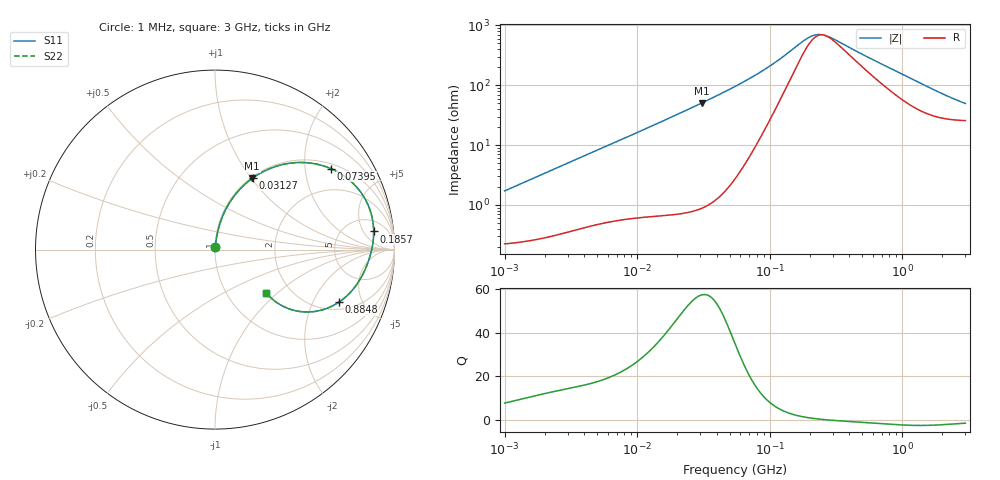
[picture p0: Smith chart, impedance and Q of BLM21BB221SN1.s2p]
! BLM21BB221SN1
# Hz S RI R 50
!Freq.(Hz) S11(Real) S11(Imag) S21(Real) S21(Imag) S12(Real) S12(Imag) S22(Real) S22(Imag)
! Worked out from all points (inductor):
!   401 points, 1 MHz to 3 GHz, reference 50 ohm
!   read as one part in series: L = 270 nH near 1.041 MHz
!   highest Q = 57.5 at 30.65 MHz (marker M1), where L = 262 nH
!   self-resonance near 257.1 MHz
!   S11 on the Smith chart (normalised r, x): 1 MHz: 1.00, +0.03; 31.27 MHz: 1.02, +1.03; 73.95 MHz: 1.15, +2.75; 185.7 MHz: 9, +9; 884.8 MHz: 2.40, -3.21; 3 GHz: 1.51, -0.85
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1000000  0.00252 0.0169  0.9975 -0.0169  0.9975 -0.0169  0.00252 0.0169
3823119  0.008 0.0627  0.992 -0.0627  0.992 -0.0627  0.008 0.0627
7858845  0.0214 0.1243  0.9786 -0.1243  0.9786 -0.1243  0.0214 0.1243
1.461624e7  0.0583 0.221  0.9417 -0.221  0.9417 -0.221  0.0583 0.221
2.181181e7  0.1164 0.3107  0.8836 -0.3107  0.8836 -0.3107  0.1164 0.3107
3.065274e7  0.2066 0.3962  0.7934 -0.3962  0.7934 -0.3962  0.2066 0.3962
3.127247e7  0.2134 0.4011  0.7866 -0.4011  0.7866 -0.4011  0.2134 0.4011
4.307715e7  0.3484 0.4665  0.6516 -0.4665  0.6516 -0.4665  0.3484 0.4665
5.477226e7  0.477 0.4854  0.523 -0.4854  0.523 -0.4854  0.477 0.4854
7.395247e7  0.6466 0.4508  0.3534 -0.4508  0.3534 -0.4508  0.6466 0.4508
1.148668e8  0.8284 0.2951  0.1716 -0.2951  0.1716 -0.2951  0.8284 0.2951
1.857042e8  0.8841 0.1012  0.1159 -0.1012  0.1159 -0.1012  0.8841 0.1012
2.094008e8  0.8826 0.0608  0.1174 -0.0608  0.1174 -0.0608  0.8826 0.0608
2.408952e8  0.8769 0.0183  0.1231 -0.0183  0.1231 -0.0183  0.8769 0.0183
2.771263e8  0.8683 -0.0203  0.1317 0.0203  0.1317 0.0203  0.8683 -0.0203
5.051982e8  0.8081 -0.1658  0.1919 0.1658  0.1919 0.1658  0.8081 -0.1658
8.005644e8  0.7174 -0.2728  0.2826 0.2728  0.2826 0.2728  0.7174 -0.2728
8.848309e8  0.6892 -0.2937  0.3108 0.2937  0.3108 0.2937  0.6892 -0.2937
1.194682e9  0.5848 -0.3393  0.4152 0.3393  0.4152 0.3393  0.5848 -0.3393
1.54974e9  0.4807 -0.3459  0.5193 0.3459  0.5193 0.3459  0.4807 -0.3459
2.177892e9  0.3599 -0.305  0.6401 0.305  0.6401 0.305  0.3599 -0.305
3e9  0.2857 -0.241  0.7143 0.241  0.7143 0.241  0.2857 -0.241
